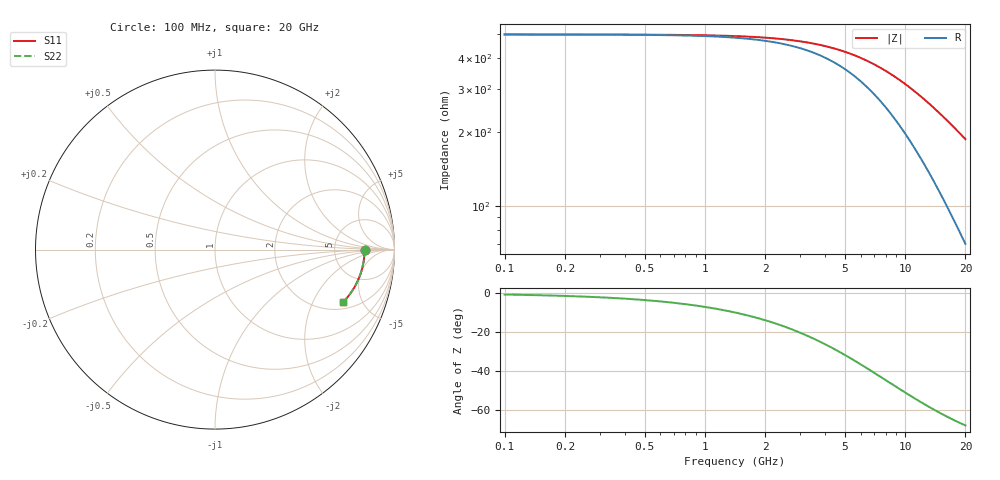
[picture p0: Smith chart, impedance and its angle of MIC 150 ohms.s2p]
! Vishay ElectroFilms Inc.
! MIC001 5000A - 500 Ohm in Series Configuration
! March 2012
# GHz S MA R 50
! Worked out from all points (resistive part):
!   233 points, 100 MHz to 20 GHz, reference 50 ohm
!   read as one part in series: R = 500 ohm at 102.3 MHz
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0.1  0.8333 -0.1  0.1667 0.6  0.1667 0.6  0.8333 -0.1
0.2436751  0.8333 -0.3  0.1667 1.4  0.1667 1.4  0.8333 -0.3
0.5937753  0.8333 -0.7  0.1671 3.5  0.1671 3.5  0.8333 -0.7
0.9375335  0.8332 -1.1  0.1678 5.5  0.1678 5.5  0.8332 -1.1
1.414214  0.833 -1.7  0.1691 8.3  0.1691 8.3  0.833 -1.7
1.860089  0.8327 -2.2  0.1709 10.8  0.1709 10.8  0.8327 -2.2
2.337309  0.8324 -2.8  0.1733 13.4  0.1733 13.4  0.8324 -2.8
2.87065  0.8319 -3.4  0.1766 16.2  0.1766 16.2  0.8319 -3.4
3.446086  0.8312 -4.1  0.1807 19.0  0.1807 19.0  0.8312 -4.1
4.330204  0.83 -5.1  0.1883 23.1  0.1883 23.1  0.83 -5.1
5.44115  0.8281 -6.4  0.1997 27.6  0.1997 27.6  0.8281 -6.4
6.099327  0.8268 -7.2  0.2072 29.9  0.2072 29.9  0.8268 -7.2
6.837118  0.8252 -8.0  0.2162 32.2  0.2162 32.2  0.8252 -8.0
8.397251  0.8211 -9.8  0.2368 36.3  0.2368 36.3  0.8211 -9.8
9.413006  0.8181 -11.0  0.2512 38.4  0.2512 38.4  0.8181 -11.0
10.55163  0.8143 -12.3  0.2679 40.3  0.2679 40.3  0.8143 -12.3
12.10121  0.8086 -14.0  0.2912 42.3  0.2912 42.3  0.8086 -14.0
13.56501  0.8026 -15.6  0.3136 43.6  0.3136 43.6  0.8026 -15.6
15.20587  0.7952 -17.4  0.3389 44.6  0.3389 44.6  0.7952 -17.4
16.66035  0.7882 -19.0  0.3612 45.2  0.3612 45.2  0.7882 -19.0
18.25396  0.78 -20.6  0.3854 45.5  0.3854 45.5  0.78 -20.6
20  0.7705 -22.4  0.4114 45.6  0.4114 45.6  0.7705 -22.4
